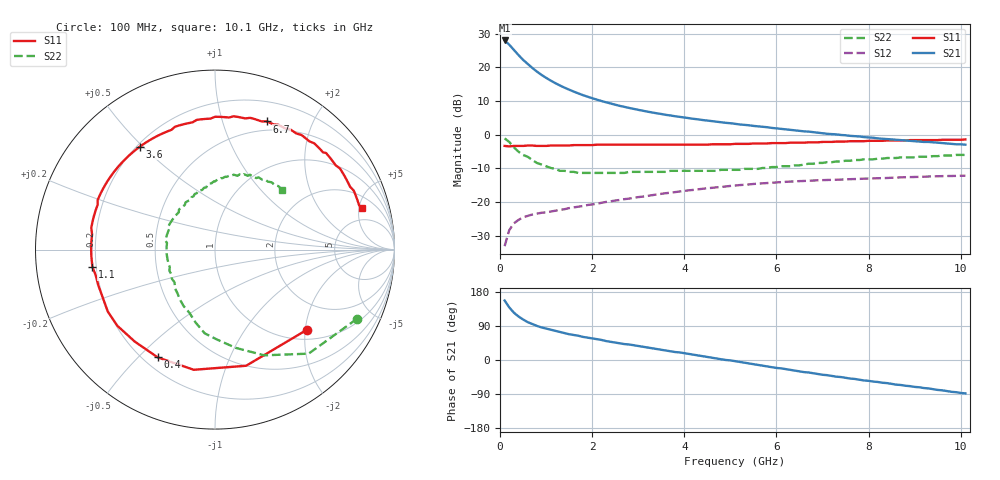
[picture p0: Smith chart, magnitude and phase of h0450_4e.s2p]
!HBFP-0450
!S and NOISE PARAMETERS at Vce=4V  Ic=15mA.  LAST UPDATED  09-04-98
# GHZ S MA R  50
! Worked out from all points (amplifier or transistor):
!   101 points, 100 MHz to 10.1 GHz, reference 50 ohm
!   highest |S21| = 28.0 dB at 100 MHz (marker M1)
!   |S21| within 3 dB of that: start of sweep to 313.8 MHz
!   unconditionally stable (mu >= 1): 2.575 GHz to end of sweep
!   at 1.7 GHz: K = 0.83, MSG = 16.8 dB, |S12| = -21.4 dB
!   at 5.1 GHz: K = 1.12, MAG = 7.1 dB, |S12| = -15.1 dB
!   at 10.1 GHz: K = 1.05, MAG = 3.3 dB, |S12| = -12.2 dB
!   lowest NFmin = 1.24 dB at 1.8 GHz
!   S11 on the Smith chart (normalised r, x): 100 MHz: 1.23, -2.05; 400 MHz: 0.26, -0.57; 1.1 GHz: 0.18, -0.07; 3.6 GHz: 0.21, +0.49; 6.7 GHz: 0.40, +1.41; 10.1 GHz: 3.14, +5.30
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0.1  0.68 -41.0  25.16 157.0  0.022 64.0  0.88 -26.0
0.2  0.67 -75.0  21.79 139.0  0.038 53.0  0.78 -48.0
0.3  0.68 -100.0  18.25 125.0  0.048 45.0  0.65 -65.0
0.4  0.68 -118.0  15.3 115.0  0.054 39.0  0.56 -78.0
0.5  0.68 -131.0  12.97 107.0  0.059 35.0  0.5 -89.0
0.6  0.69 -142.0  11.29 100.0  0.062 32.0  0.47 -97.0
0.7  0.69 -150.0  9.84 95.0  0.065 31.0  0.42 -105.0
0.8  0.68 -157.0  8.67 90.0  0.067 30.0  0.38 -112.0
0.9  0.68 -163.0  7.75 86.0  0.069 29.0  0.36 -119.0
1.1  0.69 -172.0  6.37 80.0  0.072 29.0  0.32 -131.0
1.4  0.69 176.0  5 71.0  0.078 29.0  0.29 -146.0
1.8  0.7 164.0  3.87 61.0  0.087 28.0  0.27 -162.0
2.3  0.71 152.0  3.03 50.0  0.1 27.0  0.27 -178.0
2.6  0.71 146.0  2.68 44.0  0.107 25.0  0.27 175.0
3.5  0.71 128.0  2.03 27.0  0.132 19.0  0.28 156.0
3.6  0.71 126.0  1.97 25.0  0.135 18.0  0.28 155.0
5.1  0.73 98.0  1.45 -3.0  0.175 1.0  0.3 126.0
6  0.75 81.0  1.24 -21.0  0.195 -10.0  0.33 108.0
6.7  0.77 68.0  1.11 -33.0  0.207 -20.0  0.37 95.0
6.8  0.77 66.0  1.09 -35.0  0.208 -21.0  0.37 93.0
8.5  0.82 39.0  0.85 -63.0  0.229 -43.0  0.45 68.0
10.1  0.85 16.0  0.71 -88.0  0.245 -65.0  0.5 42.0
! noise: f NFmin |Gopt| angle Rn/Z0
1.8  1.24  0.46  -169  0.06
2  1.29  0.48  -166  0.06
2.5  1.43  0.52  -153  0.08
3.5  1.71  0.6  -134  0.17
4  1.89  0.62  -122  0.28
5  2.19  0.66  -101  0.57
5.5  2.35  0.69  -90  0.82
7  2.79  0.75  -61  1.85
8  3.12  0.79  -44  2.8
10  3.7  0.82  -15  4.75
